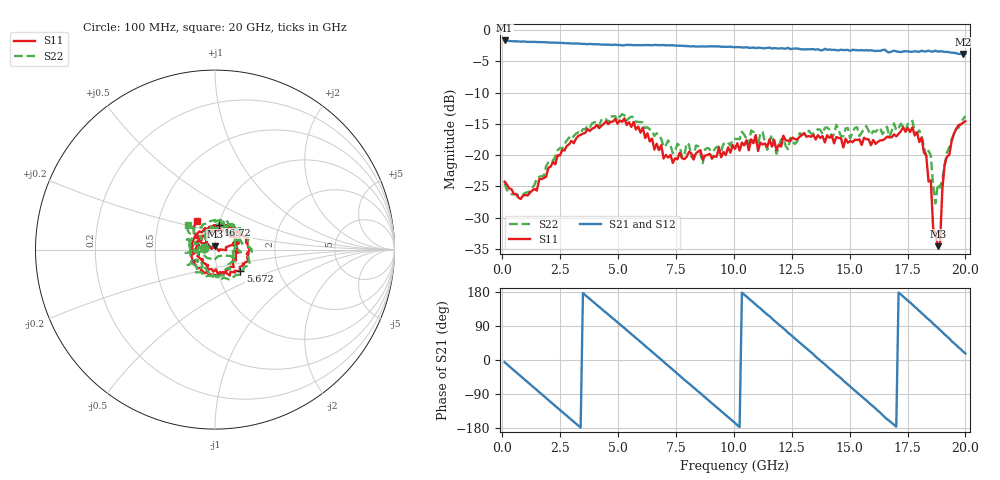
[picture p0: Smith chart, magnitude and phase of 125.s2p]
!Agilent Technologies,N5230C,MY49001569,A.09.33.09
!Agilent N5230C: A.09.33.09
!Date: Tuesday, July 21, 2015 15:12:25
!Correction: S11(Full 2 Port(1,2))
!S21(Full 2 Port(1,2))
!S12(Full 2 Port(1,2))
!S22(Full 2 Port(1,2))
!S2P File: Measurements: S11, S21, S12, S22:
# Hz S  dB  R 50
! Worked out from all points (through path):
!   201 points, 100 MHz to 20 GHz, reference 50 ohm
!   highest |S21| = -1.69 dB at 100 MHz (marker M1); lowest = -3.9 dB at 19.9 GHz (marker M2)
!   group delay of S21, straight-line fit = 147 ps
!   lowest |S11| = -34.5 dB at 18.81 GHz (marker M3), VSWR 1.04, Z = 50.1 + j1.87 ohm
!   |S11| at or under -10 dB: start of sweep to end of sweep
!   |S22| runs from -27.7 to -13.5 dB; largest |S21 - S12| = 0.028
!   S11 on the Smith chart (normalised r, x): 100 MHz: 0.89, +0.01; 5.672 GHz: 1.28, -0.32; 16.72 GHz: 1.00, +0.28; 20 GHz: 0.78, +0.26
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1e8  -24.24 173.3  -1.69 -5.7  -1.66 -5.6  -24.50 172.6
1.692e9  -23.82 140.6  -1.96 -90.0  -1.95 -89.9  -23.34 140.6
2.687e9  -19.26 106.2  -2.10 -142.2  -2.09 -141.9  -18.26 102.4
3.483e9  -16.56 70.2  -2.24 176.6  -2.25 176.6  -15.83 65.2
4.5775e9  -15.05 12.4  -2.35 119.9  -2.37 120.0  -14.89 8.6
5.672e9  -14.70 -40.5  -2.46 63.5  -2.47 63.7  -13.92 -43.9
6.7665e9  -19.21 -100.6  -2.43 6.0  -2.42 6.2  -16.86 -106.5
8.5575e9  -19.21 155.5  -2.64 -87.7  -2.59 -87.5  -19.64 162.3
1.005e10  -19.01 68.2  -2.76 -166.2  -2.74 -166.0  -17.41 78.3
1.0846e10  -18.10 34.2  -2.81 151.6  -2.89 152.2  -16.30 44.8
1.1841e10  -19.19 -24.4  -2.94 99.0  -2.90 100.1  -19.79 -11.5
1.3433e10  -16.78 -103.1  -3.08 15.4  -3.10 15.5  -16.63 -100.8
1.51245e10  -17.95 170.7  -3.17 -75.1  -3.21 -74.8  -16.39 165.9
1.67165e10  -17.16 81.5  -3.61 -160.5  -3.48 -159.7  -17.13 66.8
1.81095e10  -17.21 14.6  -3.32 124.0  -3.50 124.5  -16.90 11.9
1.85075e10  -24.05 -3.1  -3.44 102.1  -3.42 102.7  -20.08 -21.7
1.87065e10  -32.49 -20.9  -3.32 90.4  -3.48 91.4  -27.71 -65.3
1.8806e10  -34.54 85.1  -3.47 85.0  -3.46 85.5  -24.63 -94.9
1.89055e10  -34.04 167.7  -3.41 79.6  -3.42 79.9  -25.19 -107.7
1.91045e10  -21.46 153.9  -3.51 67.3  -3.59 67.8  -21.66 -169.8
1.99005e10  -14.83 127.6  -3.86 22.5  -3.92 24.8  -14.26 142.5
2e10  -14.58 121.6  -3.81 17.2  -3.81 18.6  -13.76 138.3
